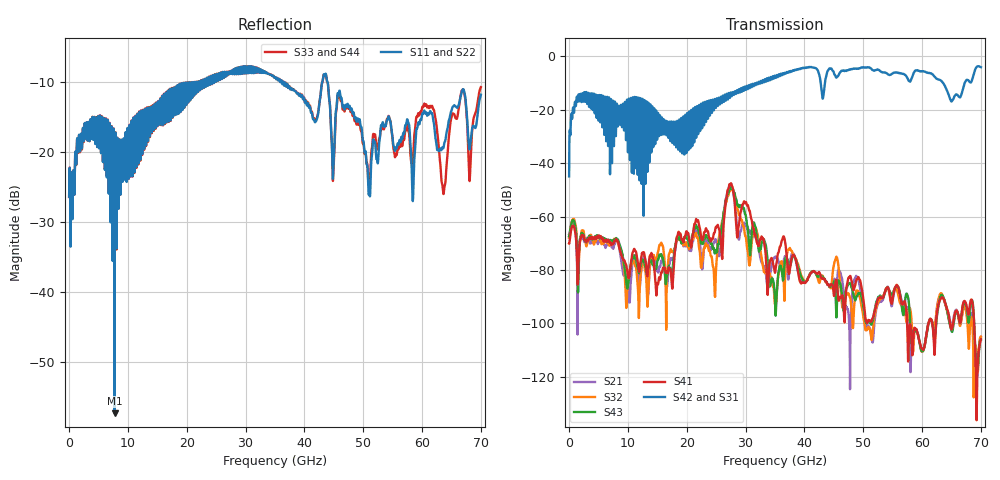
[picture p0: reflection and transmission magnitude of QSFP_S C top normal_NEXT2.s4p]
! AWR Design Environment (8415) Tue Jan 08 11:52:45 2019
! Document = 'QSFP Channel_S'
! nPorts: 4, nXvals: 7001
# HZ S DB R 50
!Freq DBS11 AngS11 DBS12 AngS12 DBS13 AngS13 DBS14 AngS14
!	DBS21 AngS21 DBS22 AngS22 DBS23 AngS23 DBS24 AngS24
!	DBS31 AngS31 DBS32 AngS32 DBS33 AngS33 DBS34 AngS34
!	DBS41 AngS41 DBS42 AngS42 DBS43 AngS43 DBS44 AngS44
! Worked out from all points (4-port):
!   7000 points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, 10 MHz to 70 GHz, reference 50 ohm
!   strongest paths, dB at 10 MHz, 17.51 GHz, 35.01 GHz, 52.51 GHz, 70 GHz:
!     S42: -44.9, -29.9, -7.3, -5.0, -4.0
!     S31: -44.9, -30.3, -7.3, -5.0, -4.0
!     S41: -70.1, -86.4, -81.0, -90.8, -106.0
!     S43: -67.5, -81.6, -91.2, -90.3, -106.0
!     S32: -68.0, -73.0, -92.7, -92.0, -104.9
!     S21: -66.8, -76.0, -75.3, -92.5, -105.1
!   lowest |S11| = -57.3 dB at 7.73 GHz (marker M1), VSWR 1.00, Z = 49.9 + j0.127 ohm
!   |S11| at or under -10 dB: start of sweep to 20.42 GHz; 36.48 GHz to 43.04 GHz (6.553 GHz wide, 16.5 % of centre); 43.96 GHz to end of sweep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
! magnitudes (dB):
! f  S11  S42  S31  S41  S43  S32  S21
! 10 MHz  -26.3  -44.9  -44.9  -70.1  -67.5  -68.0  -66.8
! 1.63 GHz  -18.3  -14.2  -14.4  -75.4  -77.0  -80.0  -73.0
! 7.73 GHz  -57.3  -18.1  -18.1  -69.1  -68.6  -68.4  -70.3
! 24.72 GHz  -9.3  -16.7  -16.7  -66.1  -73.3  -86.7  -69.4
! 27.48 GHz  -8.8  -13.5  -13.6  -47.7  -49.3  -49.8  -48.7
! 33.59 GHz  -8.6  -8.3  -8.3  -80.5  -73.3  -80.5  -84.2
! 70 GHz  -11.8  -4.0  -4.0  -106.0  -106.0  -104.9  -105.1
